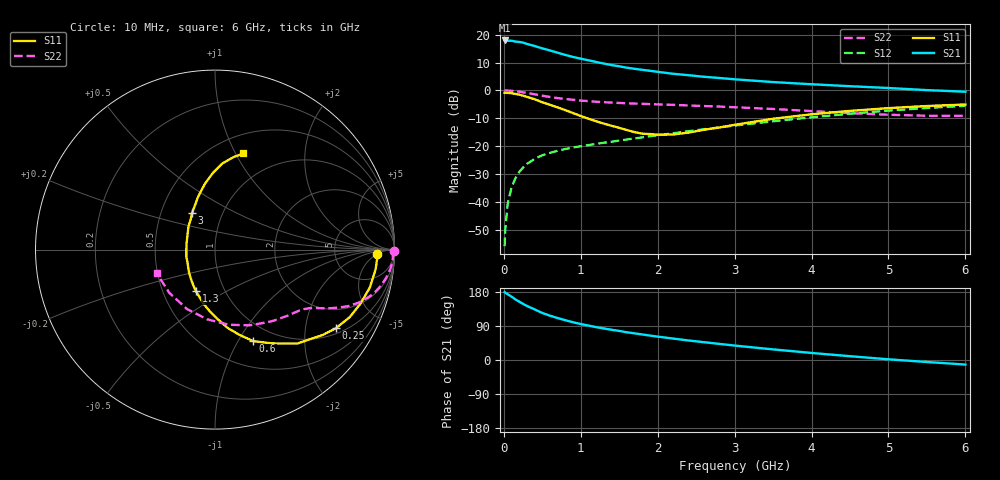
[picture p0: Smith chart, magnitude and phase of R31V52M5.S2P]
! SIEMENS Small Signal Semiconductors
! BFR181
! Si NPN RF Bipolar Junction Transistor in SOT23
! VCE = 1.5 V  IC = 2.5 mA
! Common Emitter S-Parameters:  May  1996
# GHz  S  MA  R  50
!  f  S11  S21  S12  S22
! GHz  MAG  ANG  MAG  ANG  MAG  ANG  MAG  ANG
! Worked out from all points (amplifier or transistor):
!   36 points, 10 MHz to 6 GHz, reference 50 ohm
!   highest |S21| = 17.9 dB at 10 MHz (marker M1)
!   |S21| within 3 dB of that: start of sweep to 520.8 MHz
!   unconditionally stable (mu >= 1): 1.392 GHz to 3.324 GHz
!   at 250 MHz: K = 0.27, MSG = 22.4 dB, |S12| = -27.7 dB
!   at 1.4 GHz: K = 1.00, MAG = 13.4 dB, |S12| = -18.4 dB
!   at 6 GHz: K = 0.87, MSG = 2.5 dB, |S12| = -5.5 dB
!   S11 on the Smith chart (normalised r, x): 10 MHz: 19, -5; 250 MHz: 1.19, -2.93; 600 MHz: 0.79, -1.16; 1.3 GHz: 0.73, -0.36; 3 GHz: 0.72, +0.31; 6 GHz: 0.69, +1.08
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0.01  0.9048 -1.5  7.881 178.9  0.0016 95.3  0.9959 -0.6
0.02  0.9054 -2.6  7.737 177.3  0.0034 84.4  0.9924 -1.4
0.05  0.9018 -6.9  7.788 173.5  0.0092 85.0  0.9916 -3.2
0.1  0.8884 -13.7  7.786 167.2  0.0181 80.5  0.9827 -6.3
0.15  0.8656 -20.2  7.52 160.0  0.0264 77.8  0.9665 -9.4
0.2  0.8399 -26.6  7.412 154.0  0.0344 74.6  0.9477 -12.1
0.25  0.8032 -33.1  7.198 148.0  0.0414 71.3  0.9239 -14.7
0.3  0.765 -38.5  6.828 142.7  0.0479 68.7  0.8996 -16.9
0.4  0.6957 -48.8  6.261 133.5  0.0591 64.4  0.8525 -20.3
0.5  0.6115 -58.7  5.681 124.1  0.0684 61.1  0.8045 -23.1
0.6  0.5527 -67.3  5.208 116.9  0.0757 58.4  0.7612 -25.1
0.8  0.4422 -80.8  4.326 104.9  0.0887 55.6  0.7011 -27.8
0.9  0.3916 -87.2  3.983 99.6  0.0945 55.0  0.6787 -28.8
1.1  0.3098 -101.6  3.468 90.8  0.1044 54.8  0.6409 -30.5
1.3  0.2535 -114.9  3.032 83.2  0.1151 55.1  0.6145 -32.1
1.6  0.1942 -137.9  2.555 73.1  0.1317 55.8  0.5876 -34.8
2.2  0.1618 168.6  1.988 56.6  0.1703 56.8  0.5501 -41.7
3  0.2411 121.9  1.583 38.1  0.2336 55.0  0.4985 -54.3
3.5  0.3098 107.6  1.411 28.0  0.2792 52.1  0.4641 -65.4
4.5  0.4288 91.4  1.189 10.0  0.3818 43.0  0.3908 -96.4
5.5  0.5245 78.9  1.012 -5.3  0.4833 30.3  0.3504 -136.5
6  0.5586 73.5  0.947 -12.0  0.5294 23.1  0.3506 -157.8
